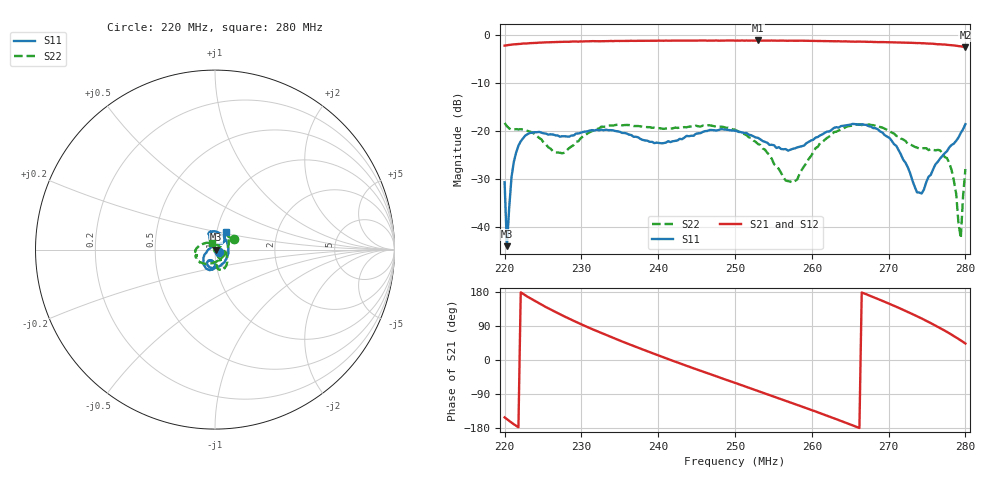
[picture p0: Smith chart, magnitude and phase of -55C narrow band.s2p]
!Agilent Technologies,E8362C,SG49020144,A.09.33.09
!Agilent E8362C: A.09.33.09
!Date: Friday, October 10, 2025 09:48:06
!Correction: S11(Full 2 Port(1,2))
!S21(Full 2 Port(1,2))
!S12(Full 2 Port(1,2))
!S22(Full 2 Port(1,2))
!S2P File: Measurements: S11, S21, S12, S22:
# Hz S  dB  R 50
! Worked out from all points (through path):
!   201 points, 220 MHz to 280 MHz, reference 50 ohm
!   highest |S21| = -1.06 dB at 253 MHz (marker M1); lowest = -2.5 dB at 280 MHz (marker M2)
!   lowest |S11| = -44.1 dB at 220.3 MHz (marker M3), VSWR 1.01, Z = 50.6 - j0.0517 ohm
!   |S11| at or under -10 dB: start of sweep to end of sweep
!   |S22| runs from -42.4 to -18.3 dB; largest |S21 - S12| = 0.0057
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2.2e8  -30.74 -33.2  -2.14 -151.4  -2.14 -151.2  -18.33 28.9
2.203e8  -44.11 -4.7  -2.06 -156.2  -2.06 -156.3  -19.00 34.2
2.209e8  -29.65 122.6  -1.93 -165.2  -1.90 -165.1  -19.71 43.5
2.221e8  -22.17 113.5  -1.77 178.5  -1.75 178.3  -19.63 49.3
2.245e8  -20.18 103.1  -1.51 149.4  -1.55 149.4  -21.45 26.4
2.275e8  -21.10 107.7  -1.34 117.8  -1.36 117.7  -24.66 -54.2
2.302e8  -20.20 111.4  -1.27 92.2  -1.26 92.3  -21.12 -115.0
2.347e8  -20.07 82.7  -1.17 53.6  -1.18 53.9  -18.70 -153.3
2.401e8  -22.52 7.0  -1.10 11.5  -1.12 11.5  -19.40 -163.1
2.446e8  -21.01 -64.8  -1.09 -21.9  -1.09 -21.7  -19.11 -163.6
2.5e8  -19.94 -110.7  -1.09 -60.4  -1.10 -60.3  -19.75 175.5
2.53e8  -21.44 -121.8  -1.06 -81.5  -1.10 -81.6  -22.74 154.6
2.575e8  -23.74 -103.7  -1.12 -113.9  -1.13 -114.1  -30.82 49.8
2.602e8  -21.82 -90.6  -1.16 -133.8  -1.16 -133.7  -24.43 -16.6
2.656e8  -18.56 -107.7  -1.32 -174.7  -1.30 -174.8  -18.62 -62.5
2.701e8  -21.42 -139.8  -1.42 148.4  -1.45 148.6  -19.96 -83.3
2.743e8  -33.09 105.9  -1.64 109.6  -1.64 109.5  -23.64 -68.5
2.776e8  -24.23 42.0  -1.97 74.2  -1.96 74.3  -25.67 -64.3
2.788e8  -22.06 48.1  -2.17 59.4  -2.18 59.4  -33.15 -78.9
2.794e8  -20.40 54.2  -2.28 51.7  -2.31 51.7  -42.44 144.6
2.797e8  -19.63 56.0  -2.38 47.7  -2.37 47.5  -33.59 118.0
2.8e8  -18.58 58.4  -2.47 43.6  -2.46 43.5  -27.97 110.6
